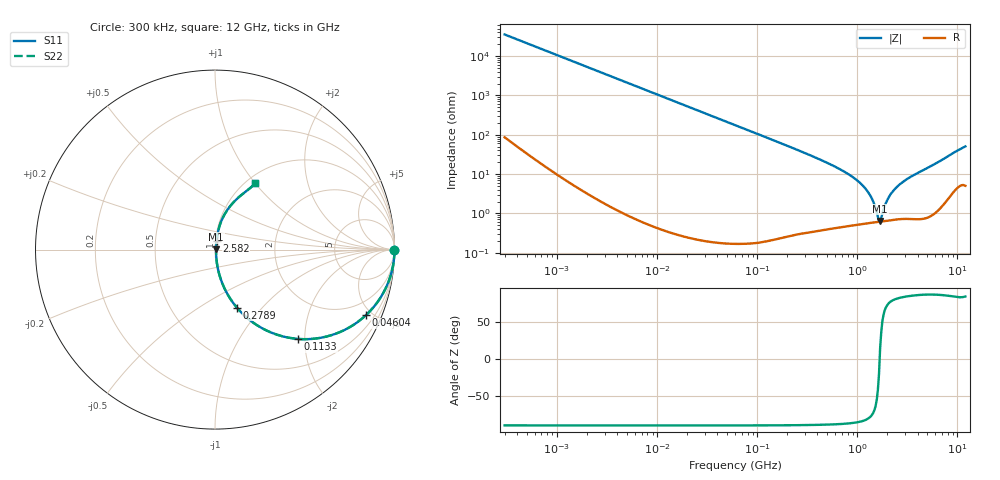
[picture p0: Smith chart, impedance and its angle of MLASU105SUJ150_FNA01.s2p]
! MLASU105SUJ150_FNA01  S-PARAMETER MODEL  ( General Type )
! Model Generated by TAIYO YUDEN Corporation (http://www.ty-top.com)
! Version 2.0
! TAIYO YUDEN Control No. 120810
! Copyright(c) 2011 TAIYO YUDEN CO.,LTD. All Rights Reserved.
! Product Description (link to TY-COMPAS)
! https://ds.yuden.co.jp/TYCOMPAS/or/detail?pn=MLASU105SUJ150JFNA01&u=M
! Products Name : Multilayer Ceramic Capacitors
! Characteristics :
!  Capacitance : 15 pF , Rated Voltage : 50V , TCC : UJ / U2J
!  Case Size : 1.0 x 0.5 / 0.039 x 0.02 [mm/inch] , Thickness : 0.5 / 0.02 [mm/inch]
!  (Conditions: Temperature = 25 degC , DC Bias Current/Voltage = 0A / 0V)
! External Node Assignments :
!  1  o---| |---o  2
! GND o---------o GND
! Frequency Range : 0.3MHz  -  12000MHz  [ 401 STEP ]
# MHz S RI R 50
! Freq[MHz].  S11 Real  S11 Imag  S21 Real  S21 Imag  S12 Real  S12 Imag  S22 Real  S22 Imag
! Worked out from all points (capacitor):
!   401 points, 300 kHz to 12 GHz, reference 50 ohm
!   read as one part in series: C = 15 pF near 316.3 kHz
!   lowest |Z| = 638 mohm at 1.69 GHz (marker M1)
!   series resonance near 1.671 GHz, so ESL is about 600 pH
!   S11 on the Smith chart (normalised r, x): 300 kHz: open; 46.04 MHz: 1.00, -4.60; 113.3 MHz: 1.00, -1.86; 278.9 MHz: 1.01, -0.74; 2.582 GHz: 1.01, +0.10; 12 GHz: 1.10, +1.01
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0.3  1 -0.00283  1.49e-05 0.00283  1.49e-05 0.00283  1 -0.00283
1.769972  0.9997 -0.0167  0.00029 0.0167  0.00029 0.0167  0.9997 -0.0167
10.44266  0.9903 -0.0977  0.00967 0.0977  0.00967 0.0977  0.9903 -0.0977
25.03118  0.947 -0.2239  0.053 0.2239  0.053 0.2239  0.947 -0.2239
46.03623  0.8406 -0.3656  0.1594 0.3656  0.1594 0.3656  0.8406 -0.3656
60  0.7563 -0.4288  0.2437 0.4288  0.2437 0.4288  0.7563 -0.4288
113.3117  0.464 -0.4977  0.536 0.4977  0.536 0.4977  0.464 -0.4977
182.544  0.2482 -0.4299  0.7518 0.4299  0.7518 0.4299  0.2482 -0.4299
278.9009  0.122 -0.3231  0.878 0.3231  0.878 0.3231  0.122 -0.3231
353.9943  0.0781 -0.2626  0.9219 0.2626  0.9219 0.2626  0.0781 -0.2626
686.4755  0.0204 -0.1252  0.9796 0.1252  0.9796 0.1252  0.0204 -0.1252
1048.836  0.0089 -0.0605  0.9911 0.0605  0.9911 0.0605  0.0089 -0.0605
1331.232  0.00651 -0.0289  0.9935 0.0289  0.9935 0.0289  0.00651 -0.0289
1441.349  0.00619 -0.0188  0.9938 0.0188  0.9938 0.0188  0.00619 -0.0188
1602.47  0.00607 -0.00553  0.9939 0.00553  0.9939 0.00553  0.00607 -0.00553
1689.663  0.00613 0.00162  0.9939 -0.00162  0.9939 -0.00162  0.00613 0.00162
1735.023  0.0062 0.00464  0.9938 -0.00464  0.9938 -0.00464  0.0062 0.00464
2088.533  0.00726 0.0261  0.9927 -0.0261  0.9927 -0.0261  0.00726 0.0261
2581.562  0.00959 0.0502  0.9904 -0.0502  0.9904 -0.0502  0.00959 0.0502
3364.605  0.0139 0.0816  0.9861 -0.0816  0.9861 -0.0816  0.0139 0.0816
6524.734  0.0514 0.1927  0.9486 -0.1927  0.9486 -0.1927  0.0514 0.1927
12000  0.2254 0.3707  0.7746 -0.3707  0.7746 -0.3707  0.2254 0.3707
